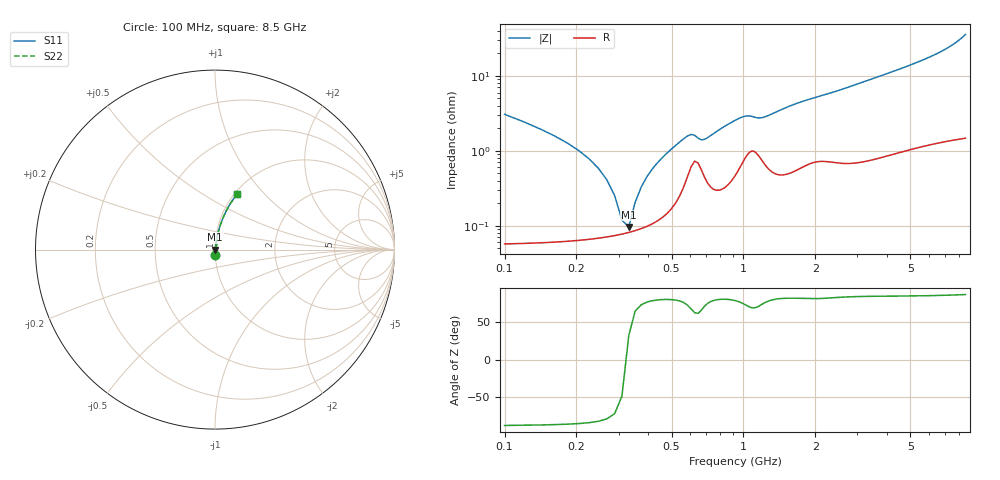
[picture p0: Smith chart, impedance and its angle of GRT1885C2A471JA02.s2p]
!Murata Part Number: GRT1885C2A471JA02
!These Parameters are Measured in Series Mode Connection
!Data Generated on Jun 19, 2026
!  o--ll--o
!Port1  Port2
!  o------o
!Operation Temp=25[degC], DC Bias Voltage=0[V]
!Freq. Start=100[MHz] Stop=9[GHz] 401[Steps]
# Hz S RI R 50
!Freq.(Hz) S11(Real) S11(Imag) S21(Real) S21(Imag) S12(Real) S12(Imag) S22(Real) S22(Imag)
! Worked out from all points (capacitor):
!   401 points, 100 MHz to 8.5 GHz, reference 50 ohm
!   read as one part in series: C = 467 pF near 142 MHz
!   lowest |Z| = 95.9 mohm at 331 MHz (marker M1)
!   series resonance near 323.4 MHz, so ESL is about 520 pH
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1e8  0.00151 -0.0306  0.9985 0.0306  0.9985 0.0306  0.00151 -0.0306
1.42e8  0.000962 -0.0193  0.999 0.0193  0.999 0.0193  0.000962 -0.0193
2.26e8  0.000715 -0.00774  0.9993 0.00774  0.9993 0.00774  0.000715 -0.00774
2.47e8  0.000712 -0.00578  0.9993 0.00578  0.9993 0.00578  0.000712 -0.00578
2.89e8  0.000741 -0.0024  0.9993 0.0024  0.9993 0.0024  0.000741 -0.0024
3.1e8  0.000771 -0.000896  0.9992 0.000896  0.9992 0.000896  0.000771 -0.000896
3.31e8  0.00081 0.000513  0.9992 -0.000513  0.9992 -0.000513  0.00081 0.000513
3.52e8  0.000859 0.00185  0.9991 -0.00185  0.9991 -0.00185  0.000859 0.00185
3.94e8  0.000994 0.00437  0.999 -0.00437  0.999 -0.00437  0.000994 0.00437
4.36e8  0.0012 0.00677  0.9988 -0.00677  0.9988 -0.00677  0.0012 0.00677
4.99e8  0.00178 0.0103  0.9982 -0.0103  0.9982 -0.0103  0.00178 0.0103
5.83e8  0.0047 0.015  0.9953 -0.015  0.9953 -0.015  0.0047 0.015
7.09e8  0.00387 0.0144  0.9961 -0.0144  0.9961 -0.0144  0.00387 0.0144
9.82e8  0.00723 0.0268  0.9928 -0.0268  0.9928 -0.0268  0.00723 0.0268
1.213e9  0.0076 0.0267  0.9924 -0.0267  0.9924 -0.0267  0.0076 0.0267
1.507e9  0.00618 0.037  0.9938 -0.037  0.9938 -0.037  0.00618 0.037
1.906e9  0.00902 0.048  0.991 -0.048  0.991 -0.048  0.00902 0.048
2.914e9  0.0123 0.0737  0.9877 -0.0737  0.9877 -0.0737  0.0123 0.0737
4.3e9  0.022 0.1129  0.978 -0.1129  0.978 -0.1129  0.022 0.1129
5.707e9  0.0371 0.1574  0.9629 -0.1574  0.9629 -0.1574  0.0371 0.1574
7.114e9  0.0629 0.2159  0.9371 -0.2159  0.9371 -0.2159  0.0629 0.2159
8.5e9  0.1232 0.3088  0.8768 -0.3088  0.8768 -0.3088  0.1232 0.3088
